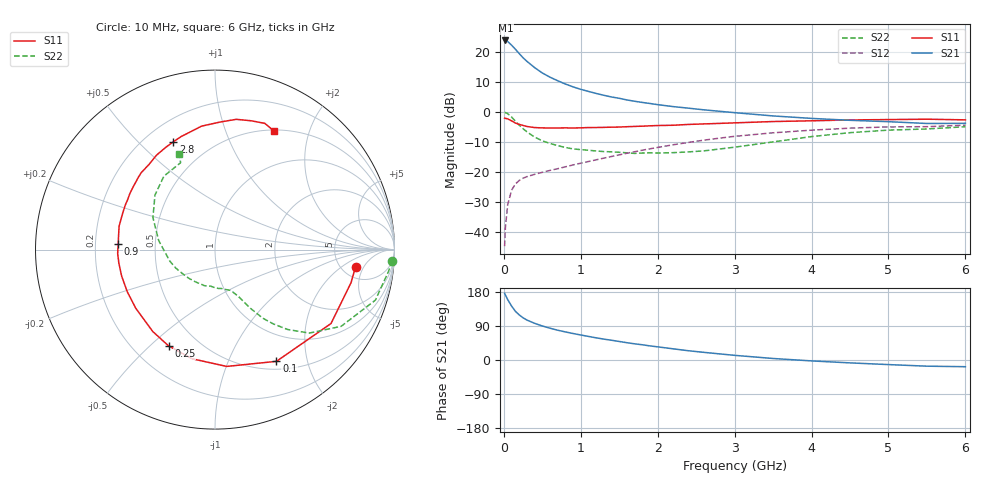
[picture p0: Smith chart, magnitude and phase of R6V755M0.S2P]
! SIEMENS Small Signal Semiconductors
! BFR193
! Si NPN RF Bipolar Junction Transistor in SOT23
! VCE = 0.75 V  IC = 5 mA
! Common Emitter S-Parameters:  May  1996
# GHz  S  MA  R  50
!  f  S11  S21  S12  S22
! GHz  MAG  ANG  MAG  ANG  MAG  ANG  MAG  ANG
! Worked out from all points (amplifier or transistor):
!   36 points, 10 MHz to 6 GHz, reference 50 ohm
!   highest |S21| = 23.7 dB at 20 MHz (marker M1)
!   |S21| within 3 dB of that: start of sweep to 153.1 MHz
!   unconditionally stable (mu >= 1): 868.7 MHz to 2.276 GHz
!   at 250 MHz: K = 0.43, MSG = 20.0 dB, |S12| = -22.0 dB
!   at 1.4 GHz: K = 1.08, MAG = 8.1 dB, |S12| = -14.8 dB
!   at 6 GHz: K = 0.99, MSG = 0.3 dB, |S12| = -4.4 dB
!   S11 on the Smith chart (normalised r, x): 10 MHz: 6.70, -3.41; 100 MHz: 0.60, -1.52; 250 MHz: 0.34, -0.57; 900 MHz: 0.30, +0.03; 2.8 GHz: 0.31, +0.64; 6 GHz: 0.51, +1.49
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0.01  0.7889 -7.0  15.21 176.1  0.0059 86.3  0.9875 -3.6
0.02  0.78 -13.7  15.35 171.5  0.012 83.4  0.9743 -7.2
0.05  0.7664 -32.5  14.74 159.5  0.0287 73.6  0.9368 -17.5
0.1  0.7105 -61.2  12.85 142.5  0.0499 61.5  0.8227 -31.3
0.15  0.6541 -84.3  10.98 128.6  0.0636 53.0  0.7018 -41.5
0.2  0.6214 -101.9  9.295 119.0  0.0727 48.1  0.6021 -47.7
0.25  0.5952 -115.8  7.917 111.4  0.0794 44.9  0.5258 -51.9
0.3  0.5733 -127.2  6.91 105.4  0.0842 43.5  0.4663 -55.1
0.4  0.5493 -143.5  5.437 96.8  0.092 42.6  0.3818 -58.9
0.5  0.5423 -154.4  4.426 89.8  0.0993 42.9  0.3312 -61.1
0.6  0.5406 -164.2  3.77 83.9  0.1068 44.1  0.2996 -62.9
0.7  0.5409 -172.0  3.29 78.6  0.114 45.8  0.2756 -65.0
0.9  0.5403 176.6  2.603 69.9  0.1316 48.7  0.2428 -69.4
1.1  0.5499 166.3  2.188 62.2  0.1501 50.6  0.2308 -74.8
1.3  0.5535 157.8  1.887 55.1  0.1709 51.7  0.2194 -80.9
1.6  0.5677 146.7  1.579 45.6  0.206 52.3  0.2091 -93.0
2.2  0.6 127.9  1.225 29.5  0.2845 48.9  0.2105 -121.5
2.8  0.644 111.2  1.025 16.2  0.3661 41.8  0.2417 -154.8
3.5  0.6919 96.2  0.857 4.0  0.4496 30.5  0.3177 170.9
4.5  0.7355 80.7  0.725 -7.6  0.5373 14.8  0.452 137.7
5.5  0.7562 68.5  0.642 -16.3  0.5685 -0.5  0.5206 111.6
6  0.7378 63.5  0.646 -17.7  0.6016 -5.0  0.5674 110.5
